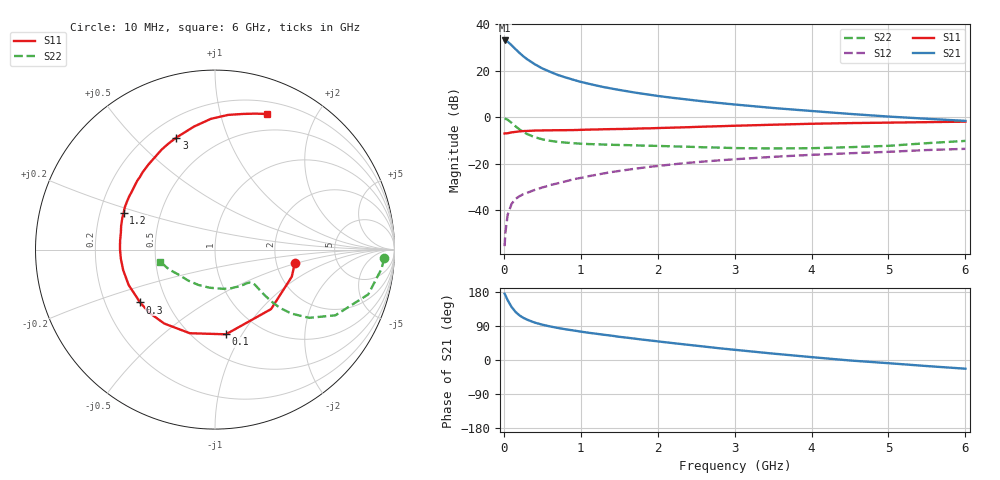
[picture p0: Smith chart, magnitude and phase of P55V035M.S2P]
! SIEMENS Small Signal Semiconductors
! BFP183
! Si NPN RF Bipolar Junction Transistor in SOT143
! VCE = 5 V  IC = 35 mA
! Common Emitter S-Parameters:  March  1996
# GHz  S  MA  R  50
!  f  S11  S21  S12  S22
! GHz  MAG  ANG  MAG  ANG  MAG  ANG  MAG  ANG
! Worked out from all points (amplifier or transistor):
!   36 points, 10 MHz to 6 GHz, reference 50 ohm
!   highest |S21| = 33.1 dB at 10 MHz (marker M1)
!   |S21| within 3 dB of that: start of sweep to 129.6 MHz
!   unconditionally stable (mu >= 1): 634.3 MHz to 5.732 GHz
!   at 250 MHz: K = 0.61, MSG = 29.7 dB, |S12| = -33.1 dB
!   at 1.4 GHz: K = 1.15, MAG = 15.6 dB, |S12| = -23.5 dB
!   at 6 GHz: K = 0.97, MSG = 6.0 dB, |S12| = -13.5 dB
!   S11 on the Smith chart (normalised r, x): 10 MHz: 2.54, -0.47; 100 MHz: 0.70, -0.85; 300 MHz: 0.35, -0.28; 1.2 GHz: 0.30, +0.18; 3 GHz: 0.30, +0.67; 6 GHz: 0.32, +1.41
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0.01  0.4509 -9.5  45.11 175.1  0.0017 81.2  0.9435 -3.0
0.02  0.4538 -19.4  44.77 171.0  0.0033 85.9  0.9344 -6.5
0.05  0.4555 -46.7  42.47 157.7  0.0081 75.6  0.8895 -16.3
0.1  0.4758 -82.6  35.72 140.2  0.0137 63.1  0.7645 -28.6
0.15  0.4867 -106.8  29.56 127.4  0.0176 55.9  0.6485 -35.9
0.2  0.4997 -124.5  24.64 118.3  0.02 53.3  0.5562 -39.9
0.25  0.5075 -135.9  20.78 111.6  0.0222 51.3  0.4895 -41.8
0.3  0.5107 -144.8  17.96 106.7  0.0238 52.2  0.4402 -42.5
0.4  0.52 -157.8  13.96 98.8  0.0275 53.0  0.3758 -42.6
0.5  0.5241 -167.3  11.3 93.2  0.031 53.4  0.3377 -42.1
0.6  0.527 -174.4  9.578 88.6  0.0349 54.8  0.3139 -41.7
0.7  0.5296 179.5  8.194 84.7  0.0382 56.4  0.2975 -41.4
0.8  0.5311 174.5  7.249 81.1  0.042 56.9  0.287 -41.4
1.1  0.5456 161.2  5.302 71.9  0.0543 57.4  0.2671 -43.2
1.2  0.5489 157.9  4.858 69.4  0.0581 57.3  0.264 -44.2
1.7  0.5717 141.5  3.421 56.4  0.0785 55.0  0.2506 -52.0
2.2  0.6019 128.0  2.628 44.5  0.0978 51.0  0.2376 -62.0
3  0.6604 109.0  1.893 26.9  0.1257 43.5  0.2188 -82.9
3.5  0.6954 99.7  1.592 16.9  0.1418 38.8  0.2146 -98.3
4.5  0.754 84.4  1.187 -1.3  0.1693 29.3  0.2287 -131.3
5.5  0.7897 73.6  0.934 -16.0  0.1985 21.2  0.2789 -156.6
6  0.8098 68.9  0.841 -23.0  0.2107 16.6  0.3122 -167.4
